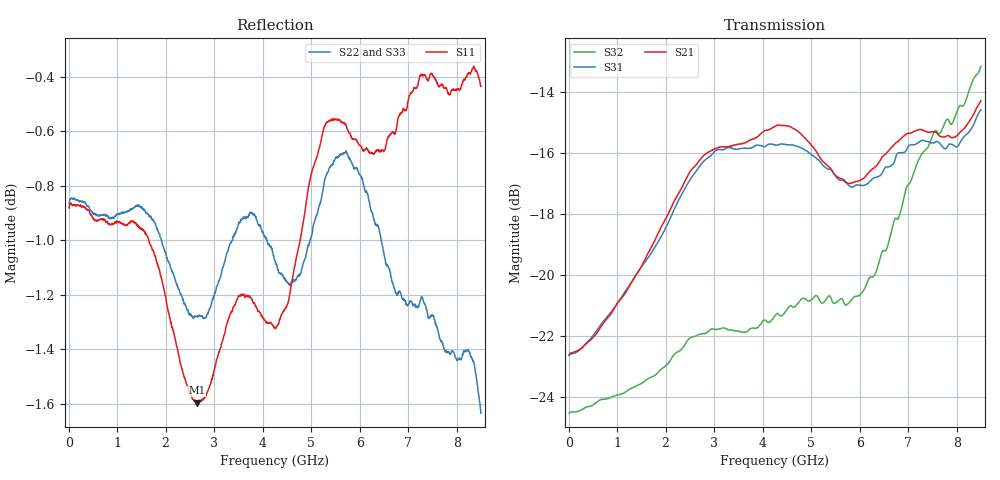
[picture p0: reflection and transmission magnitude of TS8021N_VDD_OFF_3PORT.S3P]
!Agilent Technologies,E5071C,MY46522130,B.12.04
!Date: Mon Jun 30 18:14:36 2025
!Data & Calibration Information:
!Freq	S11:SOLT4(ON)	S12:SOLT4(ON)	S13:SOLT4(ON)
!	S21:SOLT4(ON)	S22:SOLT4(ON)	S23:SOLT4(ON)
!	S31:SOLT4(ON)	S32:SOLT4(ON)	S33:SOLT4(ON)
!PortZ  Port1:50+j0  Port2:50+j0  Port3:50+j0
!Above PortZ is port z conversion or system Z0 setting when saving the data.
!When reading, reference impedance value at option line is always used.
# Hz S dB R 50
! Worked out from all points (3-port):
!   1601 points, 10 MHz to 8.5 GHz, reference 50 ohm
!   strongest paths, dB at 10 MHz, 2.132 GHz, 4.255 GHz, 6.378 GHz, 8.5 GHz:
!     S21: -22.6, -17.7, -15.1, -16.4, -14.3
!     S31: -22.6, -18.0, -15.7, -16.8, -14.6
!     S32: -24.5, -22.7, -21.3, -19.7, -13.2
!   lowest |S11| = -1.6 dB at 2.642 GHz (marker M1), VSWR 10.92, Z = 5.95 + j27.2 ohm
!   |S11| at or under -10 dB: nowhere
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1e7  -0.88 179.8  -22.62 0.1  -22.64 0.1
     -22.62 0.1  -0.87 179.8  -24.54 -0.1
     -22.65 0.1  -24.54 -0.1  -0.86 179.8
1.670856e9  -1.01 152.8  -19.19 14.0  -19.36 12.3
            -19.19 14.0  -0.91 156.5  -23.36 -2.4
            -19.36 12.3  -23.37 -2.4  -0.92 154.3
2.6419e9  -1.60 122.4  -16.35 2.3  -16.56 2.2
          -16.36 2.4  -1.28 137.1  -22.03 -9.5
          -16.57 2.2  -21.99 -9.4  -1.28 138.5
3.432531e9  -1.24 91.9  -15.74 -13.5  -15.83 -13.7
            -15.74 -13.4  -0.98 120.5  -21.83 -19.6
            -15.88 -13.8  -21.84 -19.4  -1.03 119.4
4.255e9  -1.32 66.5  -15.13 -26.4  -15.74 -26.5
         -15.13 -26.2  -1.08 113.0  -21.26 -22.8
         -15.73 -27.3  -21.34 -23.1  -1.03 111.5
5.247269e9  -0.60 40.9  -16.24 -44.9  -16.52 -43.7
            -16.29 -44.8  -0.81 92.2  -20.93 -31.5
            -16.41 -43.9  -20.92 -32.1  -0.93 95.6
6.488931e9  -0.67 37.4  -16.11 -44.5  -16.69 -43.5
            -16.09 -44.7  -1.04 97.1  -19.51 -28.8
            -16.58 -43.1  -19.20 -29.0  -1.03 97.6
6.92935e9  -0.52 32.3  -15.45 -50.1  -16.04 -47.7
           -15.42 -50.1  -1.22 90.9  -17.47 -31.7
           -15.97 -47.3  -17.35 -31.2  -1.25 95.9
7.826106e9  -0.46 35.9  -15.53 -59.8  -15.75 -56.8
            -15.43 -59.7  -1.41 71.0  -14.77 -51.4
            -15.75 -55.4  -14.91 -50.1  -1.52 76.4
8.5e9  -0.43 45.7  -14.20 -59.4  -14.32 -57.5
       -14.29 -59.3  -1.63 69.5  -13.04 -52.9
       -14.58 -58.1  -13.15 -53.5  -1.70 72.1
